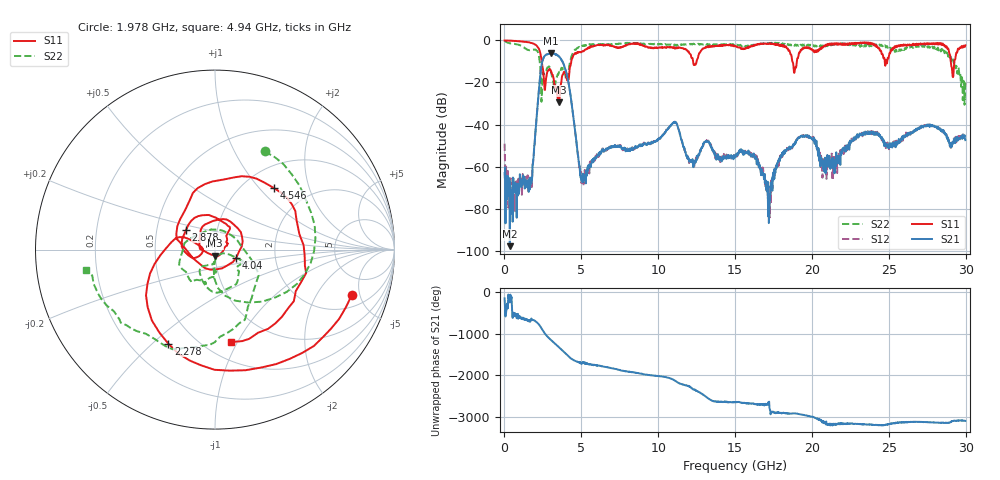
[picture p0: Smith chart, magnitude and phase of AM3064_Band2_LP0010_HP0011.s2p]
# Hz S DB R 50.0
!freq dBS11 angS11 dBS21 angS21 dBS12 angS12 dBS22 angS22
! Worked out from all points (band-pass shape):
!   1600 points, 10 MHz to 29.98 GHz, reference 50 ohm
!   highest |S21| = -6.21 dB at 3.046 GHz (marker M1); lowest = -97.9 dB at 347.4 MHz (marker M2)
!   |S21| within 3 dB of the highest: 2.495 GHz to 3.711 GHz (1.216 GHz wide, 39.2 % of centre)
!   lowest |S11| = -29.4 dB at 3.553 GHz (marker M3), VSWR 1.07, Z = 50 - j3.39 ohm
!   |S11| at or under -10 dB: 2.423 GHz to 4.344 GHz (1.921 GHz wide, 56.8 % of centre); 18.73 GHz to 19.02 GHz (292.5 MHz wide, 1.55 % of centre); 29.03 GHz to 29.26 GHz (229.4 MHz wide, 0.787 % of centre)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
!   |S22| runs from -30.6 to -0.2 dB; largest |S21 - S12| = 0.02
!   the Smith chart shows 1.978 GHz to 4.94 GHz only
!   S11 on the Smith chart (normalised r, x): 1.978 GHz: 2.96, -4.21; 2.278 GHz: 0.35, -0.56; 2.878 GHz: 0.71, +0.16; 4.04 GHz: 1.26, -0.12; 4.546 GHz: 1.36, +1.20; 4.94 GHz: 0.67, -0.94
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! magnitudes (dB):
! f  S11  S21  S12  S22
! 10 MHz  0.0  -63.2  -49.1  -0.2
! 347.4 MHz  -0.1  -97.9  -75.2  -1.3
! 1.659 GHz  -1.0  -65.2  -67.0  -4.7
! 1.978 GHz  -1.9  -47.2  -47.0  -4.2
! 2.278 GHz  -4.7  -20.3  -20.4  -9.2
! 2.878 GHz  -14.2  -6.4  -6.4  -12.4
! 3.046 GHz  -15.0  -6.2  -6.2  -15.7
! 3.553 GHz  -29.4  -7.8  -7.7  -14.7
! 4.04 GHz  -17.9  -15.8  -15.8  -18.8
! 4.546 GHz  -6.5  -40.1  -40.1  -4.8
! 4.94 GHz  -5.6  -63.1  -63.2  -2.8
! 5.015 GHz  -5.5  -66.7  -67.9  -3.0
! 10 GHz  -3.4  -46.9  -47.1  -1.8
! 15 GHz  -2.6  -55.5  -55.0  -1.9
! 16.3 GHz  -2.0  -56.3  -55.3  -2.0
! 17.18 GHz  -1.7  -76.5  -78.3  -1.5
! 18.08 GHz  -2.1  -54.8  -55.4  -1.5
! 19.99 GHz  -4.1  -46.5  -46.2  -2.1
! 20.83 GHz  -2.8  -59.6  -56.0  -2.5
! 25 GHz  -7.9  -49.9  -49.3  -3.0
! 28.56 GHz  -2.2  -43.3  -42.7  -4.7
! 29.98 GHz  -2.3  -47.4  -47.2  -19.2
